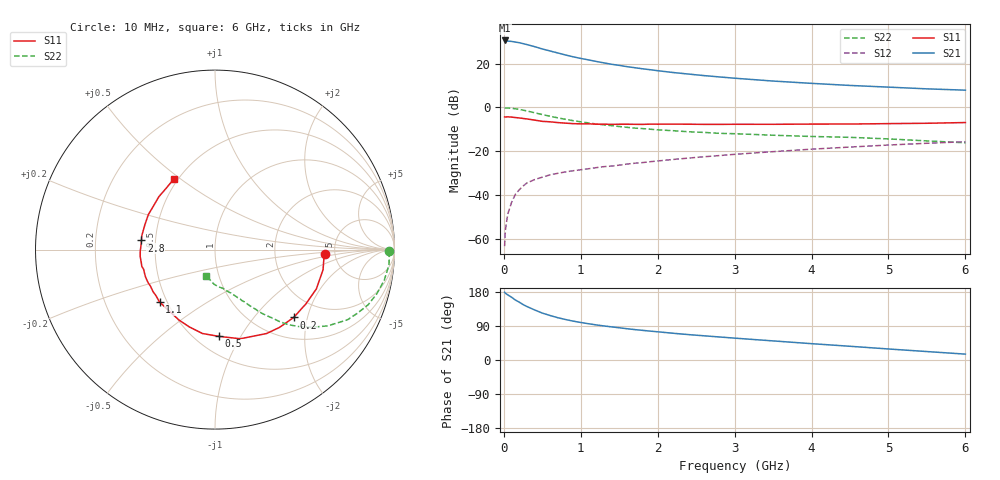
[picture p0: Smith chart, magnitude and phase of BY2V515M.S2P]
! SIEMENS Small Signal Semiconductors
! BFY420
! Si NPN RF SIEGET Grounded Emitter Transistor in MICRO-X
! VCE = 2.5 V  IC = 15 mA
! Common Emitter S-Parameters:  October  1996
# GHz  S  MA  R  50
!  f  S11  S21  S12  S22
! GHz  MAG  ANG  MAG  ANG  MAG  ANG  MAG  ANG
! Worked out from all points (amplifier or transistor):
!   36 points, 10 MHz to 6 GHz, reference 50 ohm
!   highest |S21| = 30.5 dB at 10 MHz (marker M1)
!   |S21| within 3 dB of that: start of sweep to 418 MHz
!   unconditionally stable (mu >= 1): 2.221 GHz to end of sweep
!   at 250 MHz: K = 0.24, MSG = 32.4 dB, |S12| = -35.8 dB
!   at 1.4 GHz: K = 0.86, MSG = 23.2 dB, |S12| = -26.7 dB
!   at 6 GHz: K = 1.08, MAG = 10.0 dB, |S12| = -15.6 dB
!   S11 on the Smith chart (normalised r, x): 10 MHz: 4.11, -0.32; 200 MHz: 1.45, -1.65; 500 MHz: 0.64, -0.81; 1.1 GHz: 0.46, -0.32; 2.8 GHz: 0.42, +0.05; 6 GHz: 0.48, +0.47
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0.01  0.6108 -2.3  33.5 178.8  0.0007 104.6  0.9705 -0.6
0.02  0.6087 -4.5  33.12 176.1  0.0016 78.4  0.9715 -1.7
0.1  0.6057 -21.2  31.89 165.8  0.0069 82.4  0.9583 -10.3
0.15  0.5898 -30.9  30.76 158.2  0.0106 75.3  0.9339 -15.4
0.2  0.5789 -40.8  29.77 152.7  0.0134 73.0  0.907 -19.8
0.25  0.5631 -50.3  28.4 146.3  0.0163 69.4  0.8688 -24.1
0.3  0.5489 -58.4  26.99 141.1  0.0192 67.0  0.8355 -27.9
0.4  0.5163 -74.2  24.24 132.1  0.0229 62.9  0.758 -34.1
0.5  0.484 -87.4  21.46 123.8  0.026 59.7  0.6905 -38.8
0.6  0.4727 -98.5  19.32 117.5  0.0293 57.8  0.6319 -42.7
0.7  0.4537 -108.5  17.42 111.7  0.0318 56.5  0.5824 -45.8
0.8  0.441 -117.0  15.69 106.9  0.0342 54.1  0.5387 -48.1
0.9  0.4292 -124.3  14.24 102.6  0.0364 54.1  0.5019 -49.8
1.1  0.4253 -136.6  12.1 95.7  0.0404 54.3  0.4456 -53.3
1.3  0.4172 -145.8  10.36 89.9  0.0451 54.2  0.4021 -55.7
1.6  0.4161 -158.3  8.501 82.5  0.0516 54.1  0.3538 -59.2
2.2  0.4186 -174.7  6.25 70.6  0.0657 52.9  0.2965 -64.7
2.8  0.4127 172.9  4.96 60.8  0.0805 50.8  0.2585 -69.6
3.5  0.4144 160.5  3.995 50.4  0.0989 46.9  0.234 -75.1
4.5  0.4203 144.4  3.174 36.2  0.1259 39.6  0.2094 -84.0
5.5  0.4376 128.0  2.655 22.3  0.1536 31.0  0.1739 -98.1
6  0.4546 120.5  2.478 15.5  0.1666 26.4  0.1574 -107.8
